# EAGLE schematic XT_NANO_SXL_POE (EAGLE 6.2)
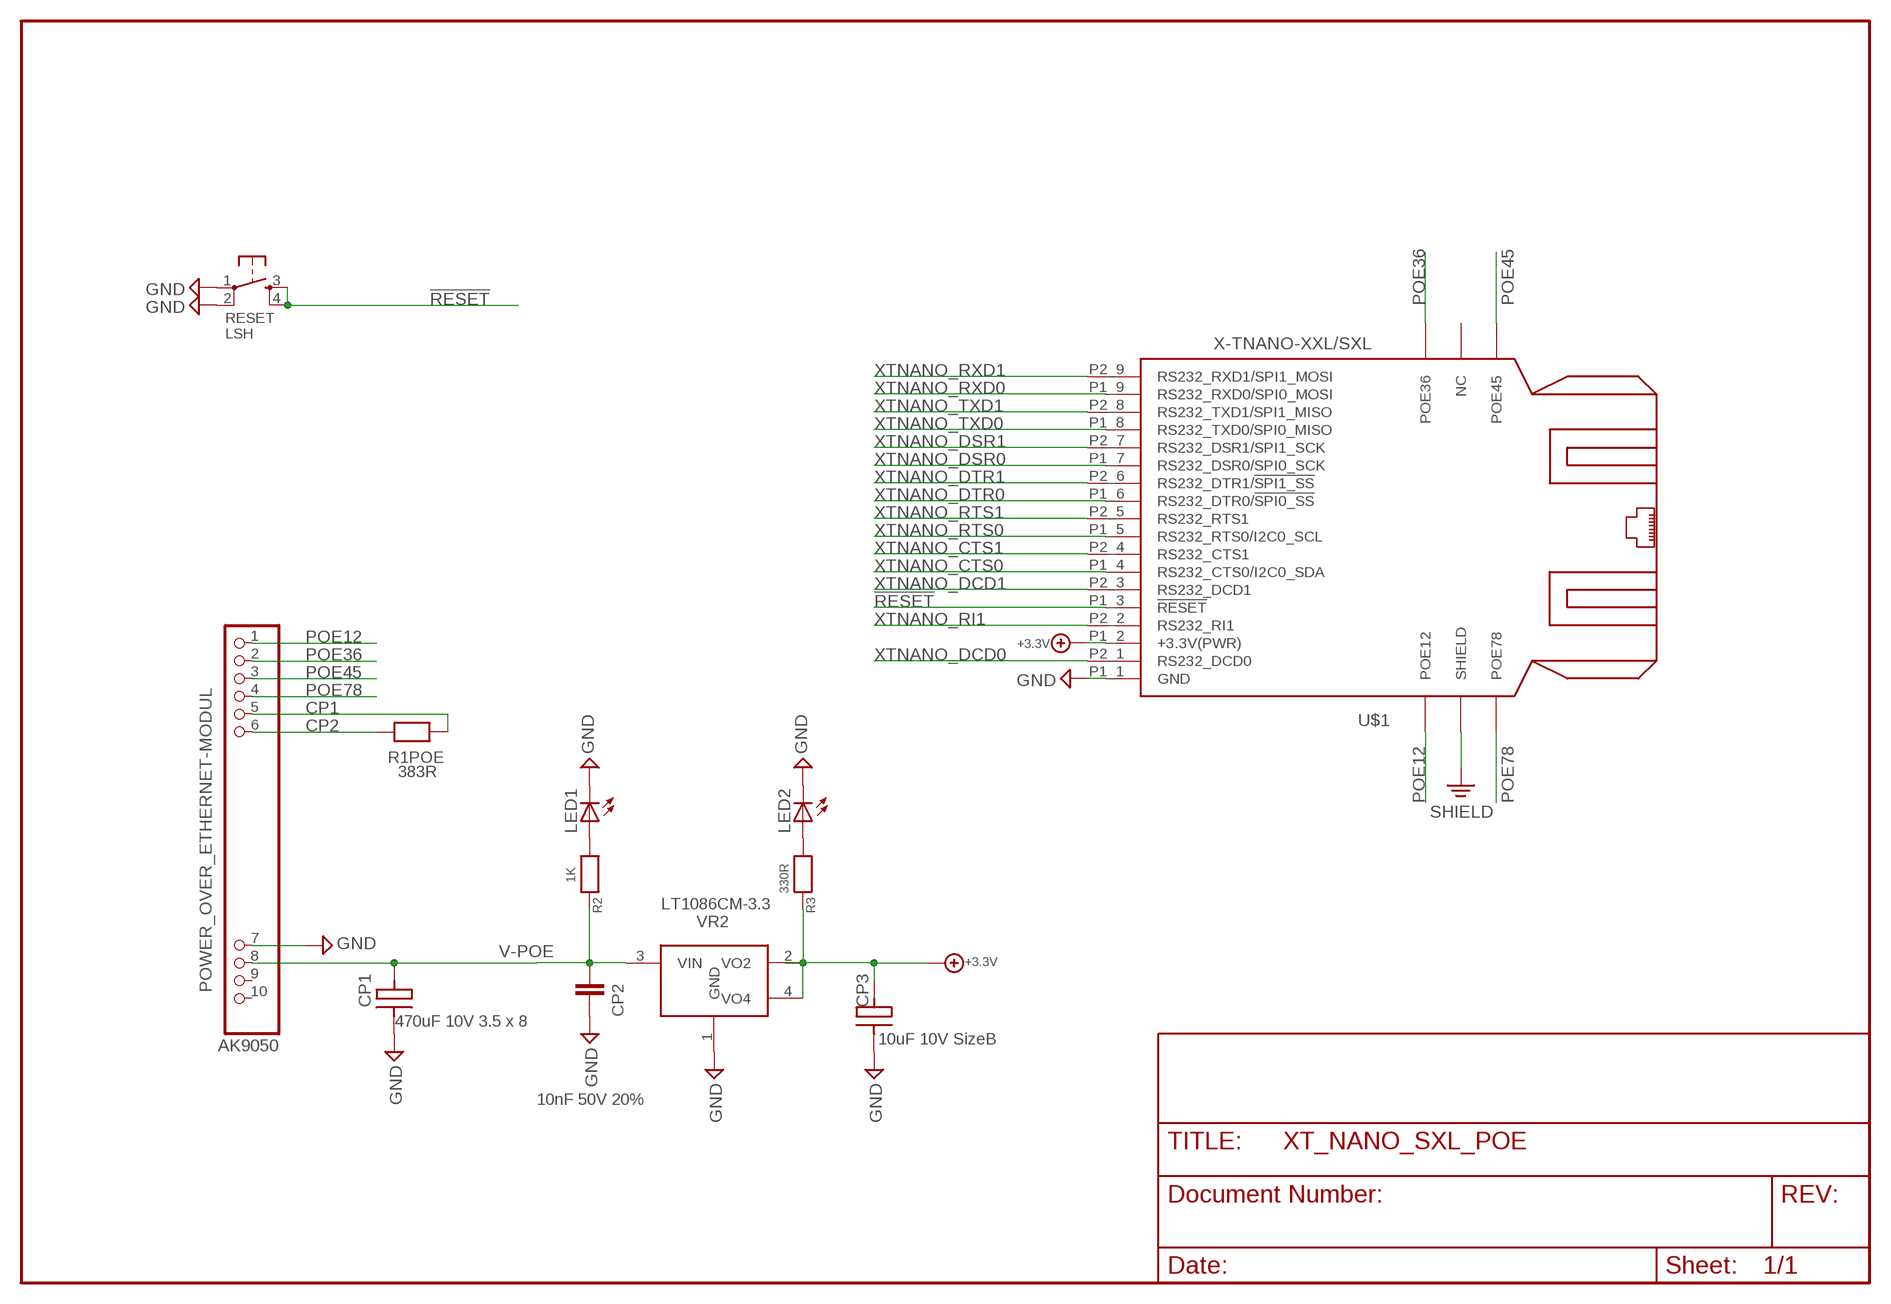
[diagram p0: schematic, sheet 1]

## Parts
CP1  470uF 10V 3.5 x 8  C3528_B  [ORCAD_X_CT3528]
CP2  10nF 50V 20%  CHIP-C-0603  [SMD-0603]
CP3  10uF 10V SizeB  C3528_B  [ORCAD_X_CT3528]
LED1  LED3MM  [LED3MM]
LED2  LED3MM  [LED3MM]
POWER_OVER_ETHERNET-MODUL  AK9050  POE_AG9000  [POE_AG9000]
R1POE  383R  CHIP-R-0603  [SMD-0603]
R2  1K  CHIP-R-0603  [SMD-0603]
R3  330R  CHIP-R-0603  [SMD-0603]
RESET  LSH  [LSH]
U$1  X-TNANO-XXL/SXL  [XT-NANO-XXL/SXL]
VR2  LT1086CM-3.3  LT1086_5.0  [DPAK_223]

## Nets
!RESET: RESET.3(S) RESET.4(S1) U$1.P1_3(!RESET)
+3.3V: CP3.1(C+) R3.2 U$1.P1_2(+3.3V(PWR)) VR2.2(VO2) VR2.4(VO4)
CP1: POWER_OVER_ETHERNET-MODUL.5(CP1) R1POE.1
CP2: POWER_OVER_ETHERNET-MODUL.6(CP2) R1POE.2
GND: CP1.2(C-) CP2.1 CP3.2(C-) LED1.K(C) LED2.K(C) POWER_OVER_ETHERNET-MODUL.7(GND) RESET.1(P) RESET.2(P1) U$1.P1_1(GND) VR2.1(GND)
N$1: CP2.2 R2.2 VR2.3(VIN)
N$37: LED1.A R2.1
N$38: LED2.A R3.1
POE12: POWER_OVER_ETHERNET-MODUL.1(VA1) U$1.POE12
POE36: POWER_OVER_ETHERNET-MODUL.2(VA2) U$1.POE36
POE45: POWER_OVER_ETHERNET-MODUL.3(VB1) U$1.POE45
POE78: POWER_OVER_ETHERNET-MODUL.4(VB2) U$1.POE78
SHIELD: U$1.SHIELD
V-POE: CP1.1(C+) POWER_OVER_ETHERNET-MODUL.8(VDC+)
XTNANO_CTS0: U$1.P1_4(RS232_CTS0/I2C0_SDA)
XTNANO_CTS1: U$1.P2_4(RS232_CTS1)
XTNANO_DCD0: U$1.P2_1(RS232_DCD0)
XTNANO_DCD1: U$1.P2_3(RS232_DCD1)
XTNANO_DSR0: U$1.P1_7(RS232_DSR0/SPI0_SCK)
XTNANO_DSR1: U$1.P2_7(RS232_DSR1/SPI1_SCK)
XTNANO_DTR0: U$1.P1_6(RS232_DTR0/!SPI0_SS!)
XTNANO_DTR1: U$1.P2_6(RS232_DTR1/!SPI1_SS!)
XTNANO_RI1: U$1.P2_2(RS232_RI1)
XTNANO_RTS0: U$1.P1_5(RS232_RTS0/I2C0_SCL)
XTNANO_RTS1: U$1.P2_5(RS232_RTS1)
XTNANO_RXD0: U$1.P1_9(RS232_RXD0/SPI0_MOSI)
XTNANO_RXD1: U$1.P2_9(RS232_RXD1/SPI1_MOSI)
XTNANO_TXD0: U$1.P1_8(RS232_TXD0/SPI0_MISO)
XTNANO_TXD1: U$1.P2_8(RS232_TXD1/SPI1_MISO)
Unconnected: POWER_OVER_ETHERNET-MODUL.9(ADJ) POWER_OVER_ETHERNET-MODUL.10(IC) U$1.FLASH(NC)

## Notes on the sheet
- 10nF 50V 20%

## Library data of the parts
CP1 CP3 = XTMACRO_AS:C3528_B
CP2 = mea-lib:CHIP-C-?: Chip capacitance
LED1 LED2 = led:LED: LED
POWER_OVER_ETHERNET-MODUL = XTMACRO:POE_AG9000: PIN HEADER
R1POE = mea-lib:CHIP-R-?: Chip resistors
R2 R3 = XTMACRO:CHIP-R-?: Chip resistors
RESET = calypso:LSH: SMD Schurter Momentary Switch
U$1 = ak-devices:X-TNANO-XXL/SXL: AK-NORD XT-NANO-XXL/SXL
VR2 = XTMACRO_AS:LT1086_5.0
